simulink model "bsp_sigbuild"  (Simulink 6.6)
settings: Solver=ode45  StartTime=0.0  StopTime=10.0  RelTol=1e-3
undefined symbols (not defined in the file or in its folder): sigbuilder_block

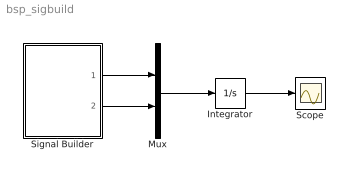
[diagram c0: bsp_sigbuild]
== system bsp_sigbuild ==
  Integrator : Integrator
  Mux : Mux  Inputs=2
  Scope : Scope
  Signal Builder : Subsystem  Tag=STV Subsys  LoadFcn=sigbuilder_block('load',[78.75 170.25 459 266.25 ]);  StartFcn=sigbuilder_block('start');  StopFcn=sigbuilder_block('stop');  ClipboardFcn=sigbuilder_block('clipboard');
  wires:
  Integrator/1 -> Scope/1
  Mux/1 -> Integrator/1
  Signal Builder/2(Signal 2) -> Mux/2
  Signal Builder/1(Signal 1) -> Mux/1

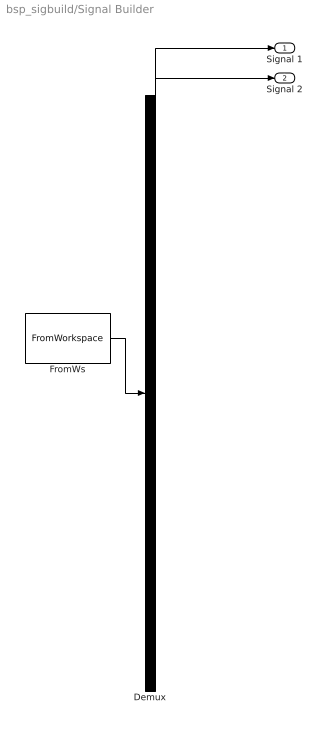
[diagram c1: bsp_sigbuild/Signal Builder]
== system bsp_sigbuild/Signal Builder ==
  Demux : Demux  Tag=STV Demux  Outputs=2
  FromWs : FromWorkspace  Tag=STV FromWs  VariableName=tuvar  SampleTime=0  OutputAfterFinalValue=Holding final value  SigBuilderData=DataTag0  VnvData=DataTag1
  Signal 1 : Outport  Tag=STV Outport
  Signal 2 : Outport  Tag=STV Outport  Port=2
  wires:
  FromWs/1 -> Demux/1
  Demux/1 -> Signal 1/1
  Demux/2 -> Signal 2/1
